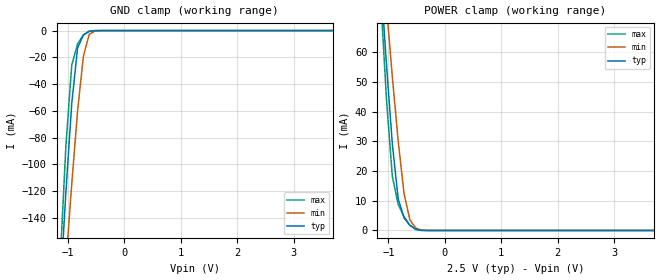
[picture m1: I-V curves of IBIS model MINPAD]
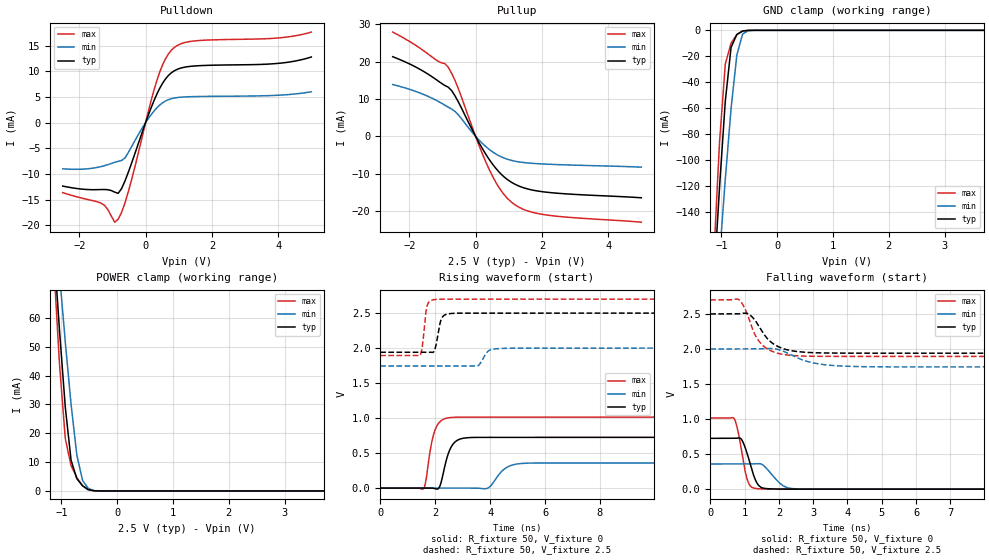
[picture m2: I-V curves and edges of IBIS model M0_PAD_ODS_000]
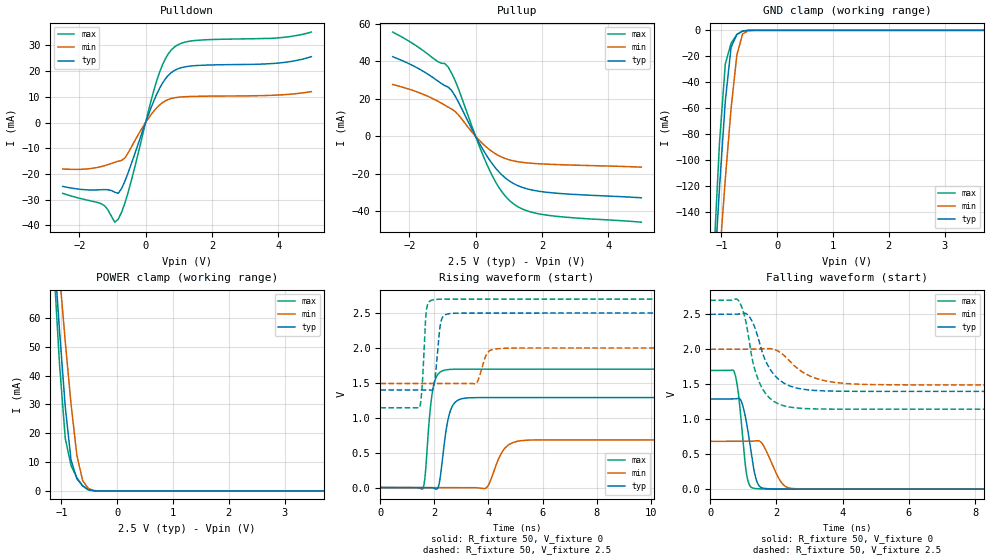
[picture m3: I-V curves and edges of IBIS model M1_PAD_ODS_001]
| Created by SiliconSmart  S-2021.06-SP5-2
[IBIS Ver]   4.0
[File Name]   as320ck_25v_rev1p2.ibs
[File Rev]   1.2
[Date]   Wed Apr 02 2025
|[Source]   Avalanche Team
|[Notes]   Generated IBIS models from Silicon Smart
|[Rev 1.0]   Initial release based on extracted netlist
|[Rev 1.1]   Updated the VCC supply values according to
|		datasheet
|[Rev 1.2]   Updated the ODS models
|[Disclaimer]   THE MODEL LIBRARIES ARE PROVIDED AS IS.
|[Copyright]   Copyright 2024, Avalanche Technology, All Rights Reserved
[Component]   AS30XX20X_BGA
[Manufacturer]  Avalanche Technology
| CONTENT :
| This file contains IBIS MODEL for PSRAM device
| AS30XX20X
| USAGE :
| The models are derived for the 2.0V to 2.7V I/O Operation.
| Temperatures for model generation: typ: 25, max: -40, min: 125
| Voltages : typ: 2.5V, min: 2.0V, max: 2.7V
| PACKAGES SUPPORTED :
| 56-ball FBGA (10mm x 10mm)
| VERIFICATION
| Errors  : 0
| Warnings: 19
| All warnings due to non-monotonic data:
[Package]
|  Design die-package: BGA
| variable   typ   min   max
R_pkg   0.72029   0.51528   1.0002
L_pkg   5.797e-9   4.155e-9   8.073e-9
C_pkg   1.116e-12   7.907e-13   1.753e-12
|Pin and Model info
[Pin]  signal_name  model_name   R_pin   L_pin   C_pin
E2   CS1#   MINPAD   0.4340	15.2000E-9	1.2600E-12
C3   CS2#   MINPAD   0.3800	13.5000E-9	1.0400E-12
D2   CLK1   MINPAD   0.4300	12.7000E-9	0.9790E-12
D1   CLK2   MINPAD   0.4480	14.6000E-9	1.1600E-12
F3   IO_0   MIOPAD   0.4010	12.4000E-9	1.2500E-12
F2   IO_1   MIOPAD   0.4050	14.2000E-9	1.1100E-12
E4   IO_2   MIOPAD   0.3780	11.8000E-9	1.2000E-12
F4   IO_3   MIOPAD   0.3700	11.8000E-9	1.2600E-12
F5   IO_4   MIOPAD   0.3710	11.1000E-9	1.1000E-12
G3   IO_5   MIOPAD   0.4050	13.8000E-9	1.1600E-12
G2   IO_6   MIOPAD   0.3830	15.2000E-9	1.0900E-12
G1   IO_7   MIOPAD   0.4480	16.4000E-9	1.0800E-12
C7   HTBSEL   MINPAD   0.1380	6.1700E-9	0.6060E-12
B7   HBP_2   MINPAD   0.1470	6.3900E-9	1.0000E-12
A6   HBP_1   MINPAD   0.1910	8.5000E-9	1.1500E-12
A5   HBP_0   MINPAD   0.2050	8.6800E-9	1.4200E-12
C4   RESET#   MINPAD   0.3410	14.1000E-9	1.6300E-12
C5   INT1#   MIOPAD   0.3080	12.5000E-9	1.2100E-12
D3   INT2#   MIOPAD   0.2120	10.3000E-9	0.8230E-12
B1   VSSIO   GND   NA   NA   NA
B5   VSSIO   GND   NA   NA   NA
B6   VSSIO   GND   NA   NA   NA
E1   VSSIO   GND   NA   NA   NA
G5   VSSIO   GND   NA   NA   NA
G6   VSSIO   GND   NA   NA   NA
A1   VSS   GND   NA   NA   NA
A3   VSS   GND   NA   NA   NA
B3   VSS   GND   NA   NA   NA
E5   VSS   GND   NA   NA   NA
E6   VSS   GND   NA   NA   NA
E7   VSS   GND   NA   NA   NA
G7   VSS   GND   NA   NA   NA
A8   VSS   GND   NA   NA   NA
A7   VCCIO   POWER   NA   NA   NA
B2   VCCIO   POWER   NA   NA   NA
B4   VCCIO   POWER   NA   NA   NA
C6   VCCIO   POWER   NA   NA   NA
F1   VCCIO   POWER   NA   NA   NA
F6   VCCIO   POWER   NA   NA   NA
G4   VCCIO   POWER   NA   NA   NA
A2   VCC   POWER   NA   NA   NA
A4   VCC   POWER   NA   NA   NA
D4   VCC   POWER   NA   NA   NA
D6   VCC   POWER   NA   NA   NA
D7   VCC   POWER   NA   NA   NA
F7   VCC   POWER   NA   NA   NA
| IOPAD
[Model Selector] MIOPAD
| Model Description
M0_PAD_ODS_000   ODS_000
M1_PAD_ODS_001   ODS_001
M2_PAD_ODS_010   ODS_010
M3_PAD_ODS_011   ODS_011
M4_PAD_ODS_100   ODS_100
M5_PAD_ODS_101   ODS_101
M6_PAD_ODS_110   ODS_110
M7_PAD_ODS_111   ODS_111
| Models and submodels in the file (9): MINPAD (Input), M0_PAD_ODS_000 (I/O), M1_PAD_ODS_001 (I/O), M2_PAD_ODS_010 (I/O), M3_PAD_ODS_011 (I/O), M4_PAD_ODS_100 (I/O), M5_PAD_ODS_101 (I/O), M6_PAD_ODS_110 (I/O), M7_PAD_ODS_111 (I/O)
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[Model] MINPAD
Model_type Input
Enable   Active-High
Vinl  =  0.7
Vinh  =  1.8
| Capacitance  typ   min   max
C_comp   1.561946e-12   1.465732e-12   1.706605e-12
| Variables   typ   min   max
[GND Clamp Reference]   0   0   0
[POWER Clamp Reference]   2.5   2   2.7
[Pulldown Reference]   0   0   0
[Pullup Reference]   2.5   2   2.7
[Temperature Range]   25   125   -40
[Voltage Range]   2.5   2   2.7
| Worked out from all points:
|   GND clamp passes 1 mA (typ) near -0.64 V on its own axis
|   POWER clamp passes 1 mA (typ) near -0.56 V on its own axis
[GND Clamp]
| Voltage   I(typ)   I(min)   I(max)
-2.5V     -1.297A    -1.146A    -1.538A
-1.138V   -195.9mA   -238.3mA   -175.2mA
-1.034V   -121.2mA   -175.1mA   -86.57mA
-931mV    -54.79mA   -114.9mA   -26.01mA
-827.6mV  -13.15mA   -60.41mA   -9.964mA
-724.1mV  -3.204mA   -19.15mA   -3.279mA
-620.7mV  -615.2uA   -2.798mA   -407.3uA
-517.2mV  -34.38uA   -319.4uA   -6.503uA
-413.8mV  -821.1nA   -24.43uA   -50.87nA
5V        0A         0A         0A
[POWER Clamp]
| Voltage   I(typ)   I(min)   I(max)
-2.5V     511mA      454.9mA    606.6mA
-1.138V   84.76mA    99.9mA     78.64mA
-1.034V   55.67mA    75.27mA    43.94mA
-931mV    29.07mA    51.7mA     18.16mA
-827.6mV  10.68mA    30.08mA    8.788mA
-724.1mV  4.238mA    12.45mA    4.618mA
-620.7mV  1.771mA    3.587mA    1.776mA
-517.2mV  465uA      837.9uA    329.7uA
-413.8mV  47.65uA    120.2uA    11.19uA
-310.3mV  1.515uA    11.72uA    116.8nA
5V        0A         0A         0A
[Model] M0_PAD_ODS_000
Model_type I/O
Enable   Active-High
Vinl  =  0.7
Vinh  =  1.8
Vmeas =  1.25
Cref  =  30e-12
| Capacitance  typ   min   max
C_comp   1.568193e-12   1.472592e-12   1.715469e-12
| Variables   typ   min   max
[GND Clamp Reference]   0   0   0
[POWER Clamp Reference]   2.5   2   2.7
[Pulldown Reference]   0   0   0
[Pullup Reference]   2.5   2   2.7
[Temperature Range]   25   125   -40
[Voltage Range]   2.5   2   2.7
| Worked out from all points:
|   slope of the pulldown table from 0 to 0.375 V, typ, clamps not added: 62.2 ohm
|   slope of the pullup table from 0 to 0.375 V, typ, clamps not added: 65.7 ohm
|   GND clamp passes 1 mA (typ) near -0.64 V on its own axis
|   POWER clamp passes 1 mA (typ) near -0.56 V on its own axis
|   falling waveform, R_fixture 50, V_fixture 0: 20-80 % time 278ps typ, 405ps min, 227ps max; typ from 0.725 V to 0 V
|   falling waveform, R_fixture 50, V_fixture 2.5: 20-80 % time 573ps typ, 848ps min, 480ps max; typ from 2.5 V to 1.94 V
|   rising waveform, R_fixture 50, V_fixture 0: 20-80 % time 317ps typ, 472ps min, 280ps max; typ from 0 V to 0.725 V
|   rising waveform, R_fixture 50, V_fixture 2.5: 20-80 % time 165ps typ, 246ps min, 130ps max; typ from 1.94 V to 2.5 V
[GND Clamp]
| Voltage   I(typ)   I(min)   I(max)
-2.5V     -1.297A    -1.146A    -1.538A
-1.138V   -195.9mA   -238.3mA   -175.2mA
-1.034V   -121.2mA   -175.1mA   -86.57mA
-931mV    -54.79mA   -114.9mA   -26.01mA
-827.6mV  -13.15mA   -60.41mA   -9.967mA
-724.1mV  -3.205mA   -19.15mA   -3.28mA
-620.7mV  -615.3uA   -2.798mA   -407.6uA
-517.2mV  -34.39uA   -319.4uA   -6.513uA
-413.8mV  -821.3nA   -24.43uA   -50.96nA
5V        0A         0A         0A
[POWER Clamp]
| Voltage   I(typ)   I(min)   I(max)
-2.5V     511mA      454.9mA    606.6mA
-1.138V   84.76mA    99.9mA     78.64mA
-1.034V   55.67mA    75.27mA    43.94mA
-931mV    29.07mA    51.7mA     18.16mA
-827.6mV  10.68mA    30.08mA    8.788mA
-724.1mV  4.238mA    12.45mA    4.618mA
-620.7mV  1.771mA    3.587mA    1.776mA
-517.2mV  465uA      837.9uA    329.7uA
-413.8mV  47.65uA    120.2uA    11.19uA
-310.3mV  1.515uA    11.72uA    116.8nA
5V        0A         0A         0A
[Pulldown]
| Voltage   I(typ)   I(min)   I(max)
-2.5V     -12.37mA   -9.009mA   -13.66mA
-1.345V   -13.05mA   -8.574mA   -15.7mA
-1.138V   -13.09mA   -8.194mA   -16.96mA
-931mV    -13.56mA   -7.743mA   -19.43mA
-827.6mV  -13.79mA   -7.541mA   -18.86mA
-517.2mV  -9.616mA   -5.796mA   -13.4mA
344.8mV   5.633mA    2.926mA    8.322mA
603.4mV   8.558mA    4.247mA    12.51mA
948.3mV   10.39mA    4.896mA    15.04mA
1.638V    11.13mA    5.111mA    16.04mA
3.99V     11.57mA    5.352mA    16.53mA
5V        12.82mA    6.029mA    17.68mA
[Pullup]
| Voltage   I(typ)   I(min)   I(max)
-2.5V     21.32mA    13.87mA    27.92mA
-1.552V   17.3mA     11.16mA    22.82mA
-827.6mV  13.18mA    7.828mA    18.54mA
-724.1mV  12.27mA    7.307mA    16.9mA
-517.2mV  9.182mA    5.729mA    12.71mA
86.21mV   -1.419mA   -832.2uA   -2.011mA
431mV     -6.452mA   -3.643mA   -9.245mA
775.9mV   -10.18mA   -5.508mA   -14.63mA
1.121V    -12.51mA   -6.533mA   -17.91mA
1.552V    -14.05mA   -7.116mA   -19.92mA
2.069V    -14.89mA   -7.424mA   -20.98mA
5V        -16.46mA   -8.263mA   -23mA
[Ramp]
dV/dt_r   0.434998/0.316698n  0.215611/0.472023n  0.608661/0.280321n
dV/dt_f   0.335983/0.573041n  0.153621/0.848322n  0.483841/0.48048n
R_load = 50
[Falling Waveform]
R_fixture = 50
V_fixture = 0
V_fixture_min = 0
V_fixture_max = 0
| Time   V(typ)   V(min)   V(max)
0s        725mV      359.4mV    1.014V
692.7ps   725.4mV    359.9mV    1.009V
780.7ps   727.4mV    359.9mV    883.5mV
897.1ps   717.9mV    360mV      593.3mV
1.087ns   490mV      360.1mV    124.4mV
1.367ns   83.45mV    363.9mV    7.307mV
1.567ns   12.57mV    331.9mV    2.275mV
2.126ns   1.009mV    48.03mV    266.1uV
2.527ns   365uV      4.584mV    159.6uV
21.88ns   -231.7nV   204.9nV    -107.4nV
[Falling Waveform]
R_fixture = 50
V_fixture = 2.5
V_fixture_min = 2
V_fixture_max = 2.7
| Time   V(typ)   V(min)   V(max)
0s        2.5V       2V         2.7V
823.1ps   2.501V     2.001V     2.707V
1.153ns   2.487V     2.001V     2.396V
1.304ns   2.409V     2.001V     2.203V
1.519ns   2.246V     2.004V     2.057V
1.886ns   2.058V     2.002V     1.951V
2.393ns   1.974V     1.908V     1.907V
3.087ns   1.946V     1.793V     1.895V
4.331ns   1.94V      1.749V     1.894V
21.88ns   1.94V      1.744V     1.894V
[Rising Waveform]
R_fixture = 50
V_fixture = 0
V_fixture_min = 0
V_fixture_max = 0
| Time   V(typ)   V(min)   V(max)
0s        3.584nV    84.08nV    3.3nV
1.569ns   -28.5uV    -123.8uV   -11.33mV
1.991ns   -8.017mV   -157.2uV   826.6mV
2.178ns   36.02mV    -171.9uV   950mV
2.497ns   512.7mV    -197.1uV   1.005V
2.897ns   699.7mV    -228.7uV   1.013V
3.862ns   724.3mV    -7.558mV   1.014V
4.611ns   724.4mV    297.4mV    1.014V
5.389ns   724.4mV    356.4mV    1.014V
21.88ns   725mV      359.4mV    1.014V
[Rising Waveform]
R_fixture = 50
V_fixture = 2.5
V_fixture_min = 2
V_fixture_max = 2.7
| Time   V(typ)   V(min)   V(max)
0s        1.94V      1.744V     1.894V
1.451ns   1.941V     1.744V     1.898V
1.701ns   1.941V     1.744V     2.597V
2.038ns   2.059V     1.745V     2.695V
2.245ns   2.432V     1.745V     2.699V
2.653ns   2.496V     1.745V     2.699V
3.54ns    2.499V     1.745V     2.699V
3.956ns   2.499V     1.964V     2.699V
4.503ns   2.499V     1.996V     2.699V
21.88ns   2.5V       2V         2.7V
[Model] M1_PAD_ODS_001
Model_type I/O
Enable   Active-High
Vinl  =  0.7
Vinh  =  1.8
Vmeas =  1.25
Cref  =  30e-12
| Capacitance  typ   min   max
C_comp   1.568193e-12   1.472592e-12   1.715469e-12
| Variables   typ   min   max
[GND Clamp Reference]   0   0   0
[POWER Clamp Reference]   2.5   2   2.7
[Pulldown Reference]   0   0   0
[Pullup Reference]   2.5   2   2.7
[Temperature Range]   25   125   -40
[Voltage Range]   2.5   2   2.7
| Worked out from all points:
|   slope of the pulldown table from 0 to 0.375 V, typ, clamps not added: 31.1 ohm
|   slope of the pullup table from 0 to 0.375 V, typ, clamps not added: 33 ohm
|   GND clamp passes 1 mA (typ) near -0.64 V on its own axis
|   POWER clamp passes 1 mA (typ) near -0.56 V on its own axis
|   falling waveform, R_fixture 50, V_fixture 0: 20-80 % time 264ps typ, 400ps min, 208ps max; typ from 1.29 V to 0 V
|   falling waveform, R_fixture 50, V_fixture 2.5: 20-80 % time 592ps typ, 885ps min, 478ps max; typ from 2.5 V to 1.4 V
|   rising waveform, R_fixture 50, V_fixture 0: 20-80 % time 286ps typ, 462ps min, 228ps max; typ from 0 V to 1.29 V
|   rising waveform, R_fixture 50, V_fixture 2.5: 20-80 % time 162ps typ, 248ps min, 124ps max; typ from 1.4 V to 2.5 V
[GND Clamp]
| Voltage   I(typ)   I(min)   I(max)
-2.5V     -1.297A    -1.146A    -1.538A
-1.138V   -195.9mA   -238.3mA   -175.2mA
-1.034V   -121.2mA   -175.1mA   -86.57mA
-931mV    -54.79mA   -114.9mA   -26.01mA
-827.6mV  -13.15mA   -60.41mA   -9.967mA
-724.1mV  -3.205mA   -19.15mA   -3.28mA
-620.7mV  -615.3uA   -2.798mA   -407.6uA
-517.2mV  -34.39uA   -319.4uA   -6.513uA
-413.8mV  -821.3nA   -24.43uA   -50.96nA
5V        0A         0A         0A
[POWER Clamp]
| Voltage   I(typ)   I(min)   I(max)
-2.5V     511mA      454.9mA    606.6mA
-1.138V   84.76mA    99.9mA     78.64mA
-1.034V   55.67mA    75.27mA    43.94mA
-931mV    29.07mA    51.7mA     18.16mA
-827.6mV  10.68mA    30.08mA    8.788mA
-724.1mV  4.238mA    12.45mA    4.618mA
-620.7mV  1.771mA    3.587mA    1.776mA
-517.2mV  465uA      837.9uA    329.7uA
-413.8mV  47.65uA    120.2uA    11.19uA
-310.3mV  1.515uA    11.72uA    116.8nA
5V        0A         0A         0A
[Pulldown]
| Voltage   I(typ)   I(min)   I(max)
-2.5V     -24.87mA   -18.07mA   -27.57mA
-1.345V   -26.16mA   -17.16mA   -31.56mA
-1.138V   -26.16mA   -16.39mA   -33.92mA
-931mV    -27.1mA    -15.47mA   -38.79mA
-827.6mV  -27.57mA   -15.06mA   -37.67mA
-517.2mV  -19.21mA   -11.59mA   -26.74mA
344.8mV   11.25mA    5.851mA    16.61mA
603.4mV   17.11mA    8.493mA    24.99mA
948.3mV   20.78mA    9.791mA    30.07mA
1.638V    22.25mA    10.22mA    32.08mA
3.99V     23.14mA    10.7mA     32.95mA
5V        25.64mA    12.06mA    35.21mA
[Pullup]
| Voltage   I(typ)   I(min)   I(max)
-2.5V     42.46mA    27.63mA    55.6mA
-1.552V   34.39mA    22.21mA    45.33mA
-827.6mV  26.27mA    15.57mA    37mA
-724.1mV  24.47mA    14.55mA    33.72mA
-517.2mV  18.31mA    11.42mA    25.35mA
86.21mV   -2.828mA   -1.659mA   -4.01mA
431mV     -12.86mA   -7.26mA    -18.44mA
775.9mV   -20.29mA   -10.98mA   -29.17mA
1.121V    -24.94mA   -13.02mA   -35.71mA
1.552V    -28.01mA   -14.18mA   -39.73mA
2.069V    -29.69mA   -14.79mA   -41.84mA
5V        -32.81mA   -16.45mA   -45.81mA
[Ramp]
dV/dt_r   0.773451/0.285827n  0.410287/0.461553n  1.01797/0.227987n
dV/dt_f   0.661206/0.592287n  0.305568/0.885073n  0.934101/0.477866n
R_load = 50
[Falling Waveform]
R_fixture = 50
V_fixture = 0
V_fixture_min = 0
V_fixture_max = 0
| Time   V(typ)   V(min)   V(max)
0s        1.289V     683.8mV    1.697V
722.1ps   1.29V      684.2mV    1.678V
850.3ps   1.298V     684.2mV    1.364V
973.2ps   1.209V     684.3mV    770.5mV
1.106ns   916.6mV    684.3mV    184.4mV
1.341ns   222mV      688.2mV    10.45mV
1.551ns   20.93mV    662mV      2.925mV
2.147ns   1.244mV    95.58mV    475.4uV
2.573ns   621uV      6.282mV    465.1uV
21.88ns   -9.112nV   105.1nV    -45.88nV
[Falling Waveform]
R_fixture = 50
V_fixture = 2.5
V_fixture_min = 2
V_fixture_max = 2.7
| Time   V(typ)   V(min)   V(max)
0s        2.5V       2V         2.7V
868.6ps   2.505V     2V         2.688V
1.048ns   2.515V     2V         2.451V
1.188ns   2.462V     2V         2.075V
1.493ns   2.083V     2.005V     1.514V
1.852ns   1.683V     2.007V     1.279V
2.373ns   1.482V     1.844V     1.175V
3.235ns   1.409V     1.578V     1.147V
4.523ns   1.399V     1.5V       1.144V
21.88ns   1.398V     1.491V     1.143V
[Rising Waveform]
R_fixture = 50
V_fixture = 0
V_fixture_min = 0
V_fixture_max = 0
| Time   V(typ)   V(min)   V(max)
0s        2.717nV    63.35nV    2.393nV
1.572ns   -650.4uV   -323.5uV   -16.16mV
1.958ns   -6.907mV   -402.9uV   1.436V
2.181ns   60.06mV    -448.8uV   1.644V
2.419ns   784.3mV    -497.9uV   1.686V
2.875ns   1.252V     -591.7uV   1.696V
3.898ns   1.289V     -10.27mV   1.696V
4.565ns   1.289V     543.2mV    1.696V
5.218ns   1.289V     671.9mV    1.696V
21.88ns   1.289V     683.8mV    1.697V
[Rising Waveform]
R_fixture = 50
V_fixture = 2.5
V_fixture_min = 2
V_fixture_max = 2.7
| Time   V(typ)   V(min)   V(max)
0s        1.398V     1.491V     1.143V
1.455ns   1.399V     1.491V     1.15V
1.545ns   1.399V     1.491V     1.432V
1.71ns    1.399V     1.491V     2.55V
1.972ns   1.441V     1.491V     2.691V
2.236ns   2.362V     1.491V     2.699V
2.57ns    2.492V     1.491V     2.699V
3.539ns   2.499V     1.49V      2.699V
4.437ns   2.499V     1.992V     2.699V
21.88ns   2.5V       2V         2.7V
